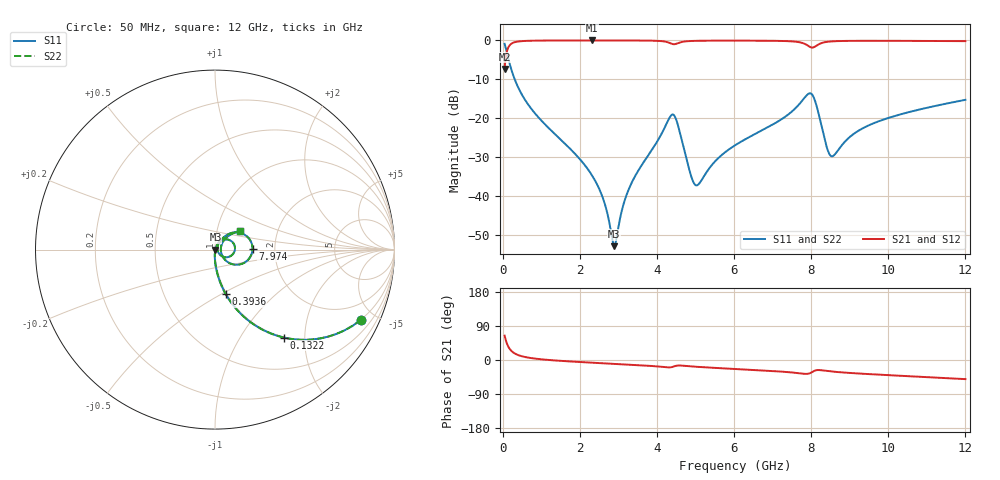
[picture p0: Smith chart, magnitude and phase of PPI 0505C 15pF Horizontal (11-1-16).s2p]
# MHz S MA R 50
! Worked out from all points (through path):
!   1601 points, 50 MHz to 12 GHz, reference 50 ohm
!   highest |S21| = -0.02 dB at 2.321 GHz (marker M1); lowest = -7.3 dB at 50 MHz (marker M2)
!   group delay of S21, straight-line fit = 13.5 ps
!   lowest |S11| = -52.8 dB at 2.896 GHz (marker M3), VSWR 1.00, Z = 50.2 - j0.0455 ohm
!   |S11| at or under -10 dB: 312 MHz to end of sweep
!   |S22| runs from -52.8 to -0.9 dB; largest |S21 - S12| = 0
!   S11 on the Smith chart (normalised r, x): 50 MHz: 0.99, -4.18; 132.2 MHz: 0.99, -1.58; 393.6 MHz: 0.99, -0.52; 7.974 GHz: 1.53, +0.02; 12 GHz: 1.28, +0.28
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50  0.9029 -25.6  0.4296 64.4  0.4296 64.4  0.9029 -25.6
132.1562  0.6216 -52.0  0.7829 38.0  0.7829 38.0  0.6216 -52.0
229.25  0.4148 -66.2  0.9093 23.7  0.9093 23.7  0.4148 -66.2
393.5625  0.2541 -76.5  0.9664 13.3  0.9664 13.3  0.2541 -76.5
864.0938  0.1116 -86.1  0.9926 3.4  0.9926 3.4  0.1116 -86.1
2044.156  0.02823 -92.1  0.9978 -5.6  0.9978 -5.6  0.02823 -92.1
2320.5  0.01837 -91.4  0.9978 -7.1  0.9978 -7.1  0.01837 -91.4
2619.25  0.008843 -85.4  0.9978 -8.7  0.9978 -8.7  0.008843 -85.4
2895.594  0.002282 -11.4  0.9975 -10.2  0.9975 -10.2  0.002282 -11.4
3283.969  0.01275 64.5  0.9968 -12.3  0.9968 -12.3  0.01275 64.5
4038.312  0.05346 58.5  0.9851 -17.1  0.9851 -17.1  0.05346 58.5
4449.094  0.1085 -6.1  0.8928 -16.7  0.8928 -16.7  0.1085 -6.1
4889.75  0.01794 -29.2  0.9822 -16.9  0.9822 -16.9  0.01794 -29.2
5024.188  0.01376 4.5  0.9869 -17.9  0.9869 -17.9  0.01376 4.5
6025  0.04494 58.8  0.9926 -23.6  0.9926 -23.6  0.04494 58.8
7705.469  0.1545 38.4  0.9449 -35.2  0.9449 -35.2  0.1545 38.4
7974.344  0.2093 1.4  0.8227 -34.6  0.8227 -34.6  0.2093 1.4
8019.156  0.2032 -9.5  0.8089 -32.2  0.8089 -32.2  0.2032 -9.5
8534.5  0.03251 -0.5  0.9711 -30.3  0.9711 -30.3  0.03251 -0.5
9161.875  0.06603 45.5  0.9867 -35.2  0.9867 -35.2  0.06603 45.5
10013.31  0.1013 45.9  0.987 -40.0  0.987 -40.0  0.1013 45.9
12000  0.1726 37.4  0.9779 -50.5  0.9779 -50.5  0.1726 37.4
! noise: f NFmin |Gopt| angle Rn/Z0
50  0.0004387  0.8809  1.165  0.0007975
1372  0.004405  0.7006  5.069  0.002875
2701  0.007614  0.6668  9.543  0.004357
4031  0.02276  0.8195  14.09  0.02601
5360  0.02066  0.7478  18.68  0.01605
6682  0.02121  0.7041  22.99  0.01352
8012  0.132  0.9359  27.67  0.433
9341  0.0292  0.7063  31.79  0.01811
1.067e+04  0.02627  0.6455  35.63  0.01279
1.2e+04  0.02743  0.6281  39.42  0.01233
